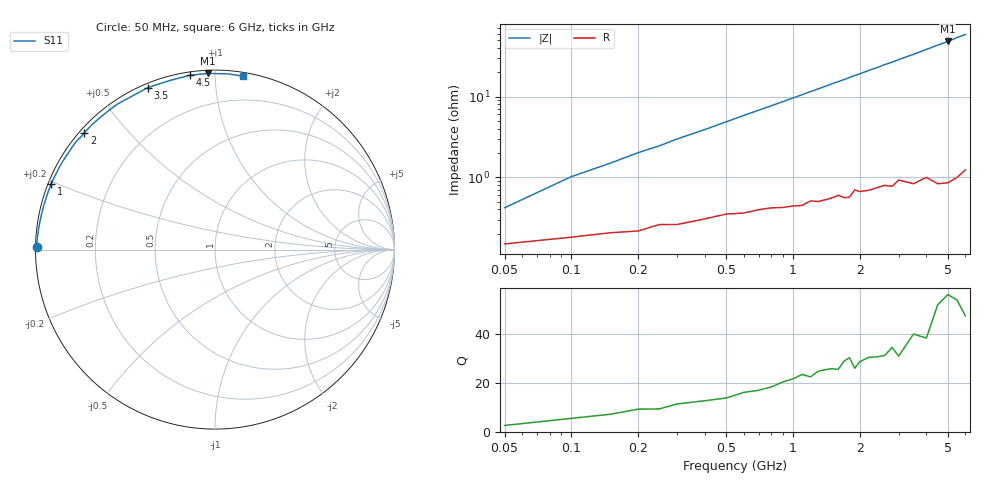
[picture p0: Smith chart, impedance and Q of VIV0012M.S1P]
! Infineon Technologies  Discrete & RF Semiconductors
! BB 804
! Si Tuning Diode in SOT23
! VR =
! S-Parameters:  July  1999
# GHz  S  MA  R  50
!  f  S11
! GHz  MAG  ANG
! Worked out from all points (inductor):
!   34 points, 50 MHz to 6 GHz, reference 50 ohm
!   read as one part to ground: L = 1.6 nH near 100 MHz
!   highest Q = 53.8 at 5 GHz (marker M1), where L = 1.53 nH
!   S11 on the Smith chart (normalised r, x): 50 MHz: 0.00, +0.01; 1 GHz: 0.01, +0.19; 2 GHz: 0.01, +0.38; 3.5 GHz: 0.02, +0.67; 4.5 GHz: 0.02, +0.86; 6 GHz: 0.02, +1.17
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0.05  0.994 179.1
0.1  0.9928 177.7
0.2  0.9914 175.4
0.25  0.9897 174.4
0.3  0.9897 173.2
0.4  0.9879 171.1
0.6  0.9858 166.7
0.8  0.9838 162.5
1  0.9831 158.3
1.1  0.9829 156.2
1.3  0.9812 152.1
1.5  0.9796 147.9
1.6  0.9783 146.0
1.7  0.9799 144.1
1.8  0.9799 142.0
1.9  0.9756 140.0
2  0.977 138.2
2.2  0.9768 134.3
2.4  0.9756 130.9
2.6  0.9748 127.1
2.8  0.9762 123.9
3  0.9725 120.4
3.5  0.9771 112.6
4  0.9751 105.1
4.5  0.9811 98.3
5  0.9823 92.3
5.5  0.9816 85.9
6  0.9794 80.9
